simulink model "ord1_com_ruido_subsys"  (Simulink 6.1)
settings: Solver=ode45  StartTime=0.0  StopTime=10.0  RelTol=1e-3
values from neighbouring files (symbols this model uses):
  Ts = 0.1    [aquisicao_dados.m]    (also in metodo_conv_cov05.m = 0.2)
undefined symbols (not defined in the file or in its folder): sigbuilder_block
libraries: simulink x1

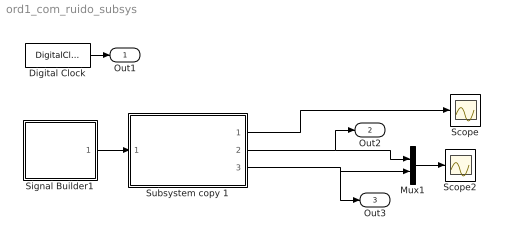
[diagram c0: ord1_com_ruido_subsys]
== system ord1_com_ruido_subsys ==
  Digital Clock : DigitalClock  SampleTime=Ts
  Mux1 : Mux  Inputs=2
  Scope : Scope
  Scope2 : Scope
  Signal Builder1 : Subsystem  Tag=STV Subsys  LoadFcn=sigbuilder_block('load');  StartFcn=sigbuilder_block('start');  StopFcn=sigbuilder_block('stop');  ClipboardFcn=sigbuilder_block('clipboard');
  Subsystem copy 1 : Subsystem
  Out1 : Outport
  Out2 : Outport  Port=2
  Out3 : Outport  Port=3
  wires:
  Subsystem copy 1/1(Saída Contínua) -> Scope/1
  Digital Clock/1 -> Out1/1
  Subsystem copy 1/3(Saída Amostrada) -> Mux1/2, Out3/1
  Subsystem copy 1/2(Entrada Amostrada) -> Out2/1, Mux1/1
  Signal Builder1/1(Signal 2) -> Subsystem copy 1/1(In1)
  Mux1/1 -> Scope2/1

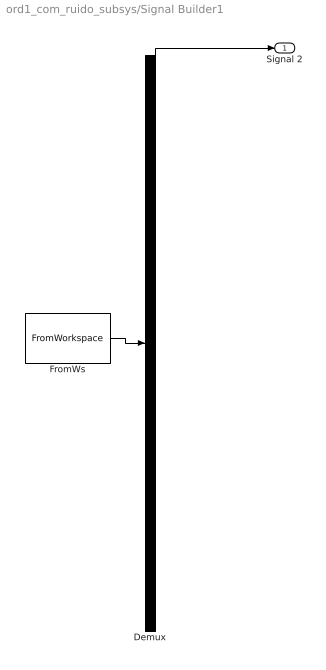
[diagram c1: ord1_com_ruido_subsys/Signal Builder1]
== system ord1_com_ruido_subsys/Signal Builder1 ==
  Demux : Demux  Tag=STV Demux  Outputs=1
  FromWs : FromWorkspace  Tag=STV FromWs  VariableName=tuvar  SampleTime=0  SigBuilderData=DataTag0  VnvData=DataTag1
  Signal 2 : Outport  Tag=STV Outport
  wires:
  FromWs/1 -> Demux/1
  Demux/1 -> Signal 2/1

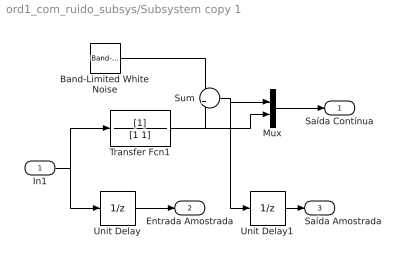
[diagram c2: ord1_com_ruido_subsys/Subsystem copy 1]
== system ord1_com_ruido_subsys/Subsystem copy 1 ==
  In1 : Inport  Port=1  LatchInput=off
  Band-Limited White Noise : simulink/Sources/Band-Limited White Noise  Cov=[0.01]  Ts=0.05  seed=[23341]
  Mux : Mux  Inputs=2
  Sum : Sum
  Transfer Fcn1 : TransferFcn  Denominator=[1 1]
  Unit Delay : UnitDelay  SampleTime=Ts
  Unit Delay1 : UnitDelay  SampleTime=Ts
  Saída Contínua : Outport
  Entrada Amostrada : Outport  Port=2
  Saída Amostrada : Outport  Port=3
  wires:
  Band-Limited White Noise/1 -> Sum/1
  Transfer Fcn1/1 -> Sum/2, Mux/2
  Sum/1 -> Mux/1, Unit Delay1/1
  Unit Delay/1 -> Entrada Amostrada/1
  Unit Delay1/1 -> Saída Amostrada/1
  In1/1 -> Transfer Fcn1/1, Unit Delay/1
  Mux/1 -> Saída Contínua/1
